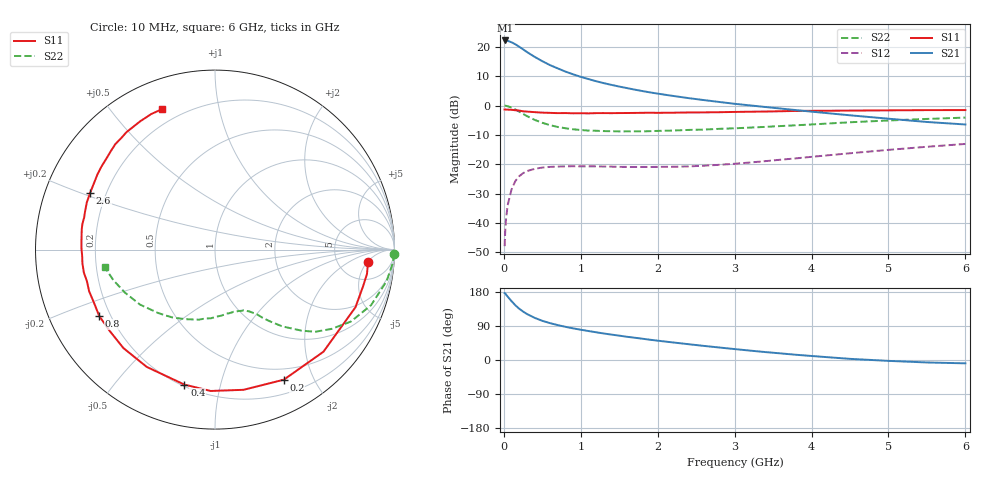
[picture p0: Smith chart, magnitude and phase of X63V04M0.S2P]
! SIEMENS Small Signal Semiconductors
! BFP193W
! Si NPN RF Bipolar Junction Transistor in SOT343
! VCE = 3 V  IC = 4 mA
! Common Emitter S-Parameters:  April 1994
# GHz  S  MA  R  50
!  f  S11  S21  S12  S22
! GHz  MAG  ANG  MAG  ANG  MAG  ANG  MAG  ANG
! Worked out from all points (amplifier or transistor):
!   40 points, 10 MHz to 6 GHz, reference 50 ohm
!   highest |S21| = 22.2 dB at 20 MHz (marker M1)
!   |S21| within 3 dB of that: start of sweep to 248.9 MHz
!   unconditionally stable (mu >= 1): 1.769 GHz to 4.504 GHz
!   at 200 MHz: K = 0.28, MSG = 22.1 dB, |S12| = -24.1 dB
!   at 1.5 GHz: K = 0.88, MSG = 13.7 dB, |S12| = -20.9 dB
!   at 6 GHz: K = 0.91, MSG = 3.3 dB, |S12| = -13.1 dB
!   S11 on the Smith chart (normalised r, x): 10 MHz: 10, -5; 200 MHz: 0.36, -1.60; 400 MHz: 0.21, -0.78; 800 MHz: 0.16, -0.26; 2.6 GHz: 0.14, +0.21; 6 GHz: 0.13, +0.68
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0.01  0.8554 -4.5  12.83 176.6  0.004 88.5  0.9978 -1.3
0.02  0.8576 -9.1  12.86 174.8  0.0081 83.1  0.9927 -4.4
0.05  0.8504 -13.6  12.67 167.2  0.02 79.0  0.9722 -10.4
0.1  0.846 -22.3  11.96 155.3  0.0371 67.7  0.9231 -19.6
0.15  0.8299 -43.3  11.07 144.3  0.0516 58.2  0.8566 -27.9
0.2  0.82 -62.1  10.03 135.3  0.0624 50.7  0.7858 -34.2
0.25  0.7972 -78.5  9.085 127.9  0.0702 44.5  0.7216 -39.4
0.3  0.788 -91.7  8.172 121.4  0.0762 39.6  0.661 -43.1
0.4  0.7712 -102.8  6.759 111.3  0.0832 32.2  0.57 -48.7
0.5  0.7562 -120.2  5.7 103.4  0.0876 27.4  0.5078 -52.3
0.6  0.7493 -132.9  4.888 97.3  0.0899 23.7  0.4627 -55.1
0.7  0.7414 -142.5  4.299 92.1  0.0909 21.5  0.4312 -57.0
0.8  0.7437 -150.2  3.791 87.6  0.0918 19.9  0.4099 -59.1
1.1  0.735 -166.1  2.826 76.4  0.0918 17.3  0.374 -64.7
1.3  0.7427 -174.1  2.405 69.9  0.0911 16.7  0.3665 -68.9
1.6  0.7452 176.9  1.983 61.3  0.0898 18.1  0.3625 -75.1
2.2  0.7542 163.9  1.457 46.3  0.0904 24.1  0.3743 -88.9
2.6  0.764 155.6  1.238 37.2  0.0942 29.6  0.3886 -98.5
3.2  0.7838 143.8  1.005 24.8  0.1068 36.5  0.4204 -112.7
4.5  0.8193 127.0  0.681 3.0  0.1535 41.8  0.5183 -143.8
5.5  0.8347 115.2  0.524 -6.5  0.198 38.8  0.5911 -163.2
6  0.8363 110.6  0.475 -8.8  0.2213 36.6  0.6223 -170.9
